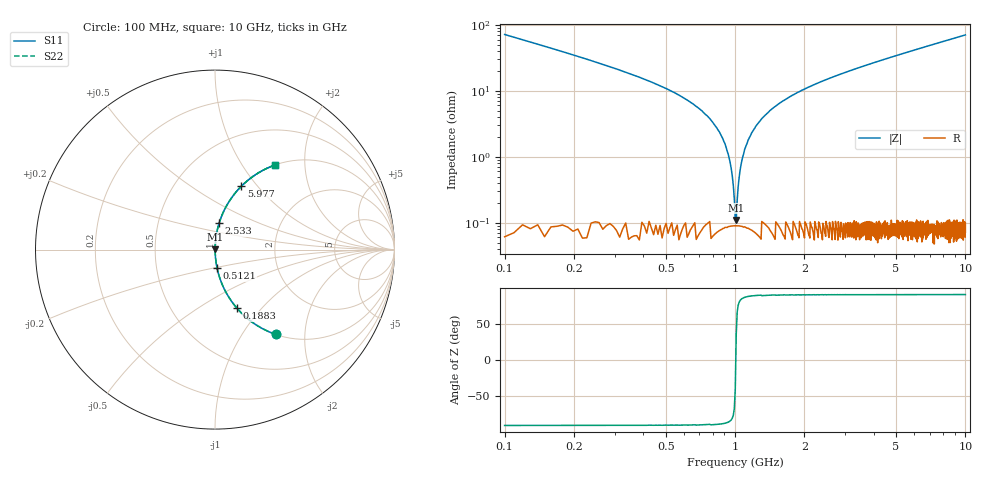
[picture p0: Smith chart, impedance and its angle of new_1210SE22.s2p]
!	AVX	Thin	Film	Operation	Date:	April 2007
!	Description:	Accu-P®	"Series,"	Thin	"Film,"	"SMD,"	RF	Capacitor
!	Part	Number:	12101J200FBT
!	100	MHz	-	5.05	GHz
!	Serial	Measurements
#	MHZ	S	MA	R	50
!	S11	S21	S12	S22
!	dB	Phase	dB	Phase	dB	Phase	dB	Phase
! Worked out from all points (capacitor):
!   1010 points, 100 MHz to 10 GHz, reference 50 ohm
!   read as one part in series: C = 22 pF near 149.1 MHz
!   lowest |Z| = 110 mohm at 1.012 GHz (marker M1)
!   series resonance near 1.008 GHz, so ESL is about 1.1 nH
!   S11 on the Smith chart (normalised r, x): 100 MHz: 1.00, -1.43; 188.3 MHz: 1.00, -0.74; 512.1 MHz: 1.00, -0.21; 2.533 GHz: 1.00, +0.30; 5.977 GHz: 1.00, +0.83; 10 GHz: 1.00, +1.41
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100  0.582 -54.3  0.813 35.6  0.813 35.6  0.582 -54.3
188.305  0.347 -69.5  0.937 20.3  0.937 20.3  0.347 -69.5
512.091  0.104 -83.6  0.994 6.0  0.994 6.0  0.104 -83.6
718.137  0.05 -86.2  0.998 2.8  0.998 2.8  0.05 -86.2
835.877  0.027 -86.8  0.999 1.5  0.999 1.5  0.027 -86.8
914.371  0.014 -85.9  0.999 0.8  0.999 0.8  0.014 -85.9
933.994  0.011 -85.2  0.999 0.6  0.999 0.6  0.011 -85.2
973.241  0.0051 -80.7  0.999 0.3  0.999 0.3  0.0051 -80.7
1012.488  0.00102 38.6  0.999 -0.0  0.999 -0.0  0.00102 38.6
1041.923  0.00482 80.2  0.999 -0.3  0.999 -0.3  0.00482 80.2
1081.169  0.01 84.9  0.999 -0.6  0.999 -0.6  0.01 84.9
1110.605  0.014 85.9  0.999 -0.8  0.999 -0.8  0.014 85.9
1228.345  0.029 86.8  0.999 -1.6  0.999 -1.6  0.029 86.8
1463.826  0.055 86.0  0.998 -3.1  0.998 -3.1  0.055 86.0
1758.176  0.084 84.7  0.996 -4.8  0.996 -4.8  0.084 84.7
2533.3  0.15 81.1  0.988 -8.6  0.988 -8.6  0.15 81.1
3406.541  0.216 77.3  0.976 -12.5  0.976 -12.5  0.216 77.3
5054.906  0.326 70.8  0.944 -19.1  0.944 -19.1  0.326 70.8
5977.205  0.382 67.4  0.923 -22.4  0.923 -22.4  0.382 67.4
6703.271  0.422 64.9  0.906 -25.0  0.906 -25.0  0.422 64.9
8351.635  0.505 59.6  0.862 -30.3  0.862 -30.3  0.505 59.6
10000  0.576 54.8  0.817 -35.2  0.817 -35.2  0.576 54.8
